ORGANIZATION_BLOCK MAIN:OB1
TITLE= Avviatore Stella-Triangolo per M.A.T.
// Simulatore: 02
// Versione: 1.0
// Data: 28/02/2002
//
//----------- Descrizione del Controllo -----------------
// Il pulsante SB1 (I0.4) inserisce il contattore KM3
// predisposto per il collegamento a Stella del Motore e nello
// stesso tempo fa partire il temporizzatore T32 ritardato
// all'eccitazione.
// Il contatto NA di KM3 (KM3a) da il consenso all'eccitazione
// del contattore principale di linea KM1 e il motore funziona
// quindi a stella.
// Trascorso il tempo di ritardo (5 s) il contatto del temporizzatore
// T32 disinserisce il contattore di stella KM3.
// La disinserzione di KM3 da il consenso all'eccitazione del
// contattore KM2 e il motore marcia regolarmente a triangolo.
// Il pulsante SB2 (I0.5) può arrestare in qualsiasi momento
// la marcia del motore.
// I contattori KM3 e KM2 non possono essere inseriti conteporaneamente
// e quindi è necessario creare un interblocco elettrico hardware oltre
// a quello software gestito dal PLC.
// Il motore è protetto da un relè termico FR.
// Per motivi di sicurezza  un contatto NC del Relè Termico
// FR viene collegato in hardware a monte della bobina dei contattori,
// se inteviene la protezione le bobine dei contatori vengono
// disinserita direttamente via hardware senza l'intervento
// del controllore programmabile.
// Un contatto NC di RT viene però riportato anche su un
// ingresso (I0.0) del PLC per disattivare le uscite in caso di
// intervento dello stesso e segnalare mediante la lampada
// HL4 il suo intervento.
// Le segnalazioni sono affidate a tre lampade che segnalano:
// HL3: lo stato di motore Fermo
// HL2: Lo Stato di motore in marcia a triangolo quando è
//      accesa in continuità e lo stato di marcia a stella
//      quando lampeggia.
// HL4: L'intervento del relè termico.
//------------- Particolarità Programma ----------------
// Il presente programma effetua anche un'interrogazione dello
// stato dei contattori verificando se dopo un normale tempo
// di commutazione lo stato effettivo del contattore corrisponde
// al segnale di uscita del PLC.
// Se si verifica una discordanza fra i segnali questo
// significa che si è verificato un guasto e il motore deve
// essere immediatamente disattivato e una lampada HL1
// segnala la presenza del guato.
// Prima di riavviare il motore il guasto deve essere tacitato
// (resettato) mediante il pulsante SB3.

BEGIN
NETWORK 1 //Merker attivazione teleruttore stella
//
LD I0.1
AN I0.2
LD I0.2
A I0.4
OLD
A I0.5
A I0.0
AN Q0.2
= M0.0

NETWORK 2 //Attivazione Contattore Stella
//
LD M0.0
AN M1.0
AN T32
= Q0.1

NETWORK 3 //Temporizzatore Stella
//
LD M0.0
TON T32 +50

NETWORK 4 //SET Contattore di Linea
//
LD I0.1
A I0.4
S Q0.0 1

NETWORK 5 //RESET Contatore di Linea
//
LD I0.3
ED
ON I0.0
ON I0.5
O M1.0
R Q0.0 1

NETWORK 6 //Gestione Contattore Triangolo
//
LD I0.2
AN I0.4
= Q0.2

NETWORK 7 //Test Commutazione contattori
//
LD Q0.0
AN I0.2
LDN Q0.0
A I0.2
OLD
LD Q0.1
AN I0.4
OLD
LDN Q0.1
A I0.4
OLD
LD Q0.2
AN I0.3
OLD
LDN Q0.2
A I0.3
OLD
TON T33 +2

NETWORK 8 //SET Merker Guasto
//
LD T33
S M1.0 1

NETWORK 9 //RESET Merker Guasto
//
LDN I0.6
R M1.0 1

NETWORK 10 //Segnalazione Motore Fermo
//
LDN Q0.0
= Q0.3

NETWORK 11 //Segnalazione Marcia motore (Lampeggio a stella)
//
LD Q0.0
A Q0.2
LD SM0.5
A Q0.1
OLD
= Q0.4

NETWORK 12 //Segnalazione intervento relè termico
//
LDN I0.5
= Q0.6

NETWORK 13 //Segnalazione Guasto
//
LD M1.0
= Q0.5

END_ORGANIZATION_BLOCK

